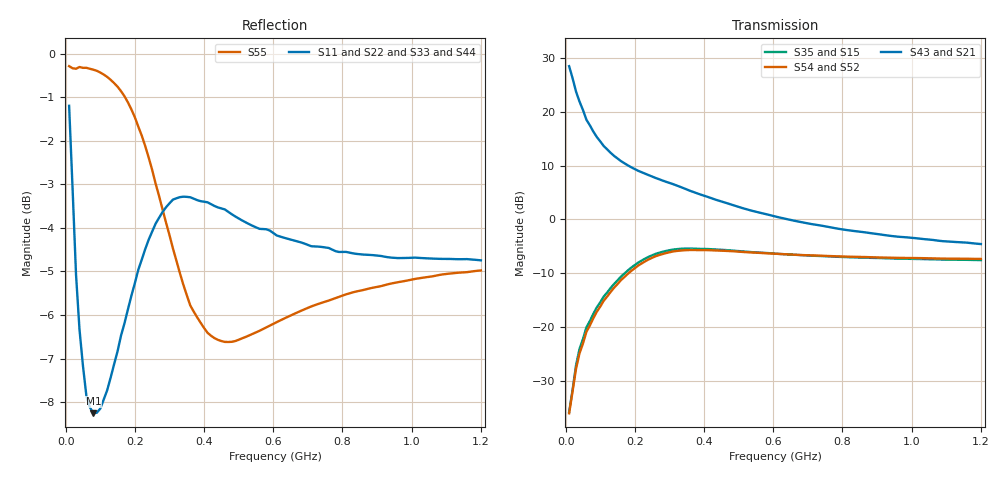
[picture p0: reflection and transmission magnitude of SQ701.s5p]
!  POLYFET RF DEVICES
!  S PARAMETERS FOR
!  SQ701 (EACH SIDE)
!  VDS=28, IDQ=200MA
! S1A1Die, Vds=28Vdc, Idq=200ma, Vgsth=2.60Vdc
! Date: Thu Jul 23 11:46:25 1998
!AWR Design Environment (2053) Wed Feb 04 15:37:27 2004
!freq-unit  param-type  data-format  keyword  impedance-ohms
# MHz  S  MA  R  50
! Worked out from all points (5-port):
!   120 points, 10 MHz to 1.2 GHz, reference 50 ohm
!   strongest paths, dB at 10 MHz, 310 MHz, 610 MHz, 910 MHz, 1.2 GHz:
!     S43: 28.5, 6.6, 0.5, -2.8, -4.6
!     S21: 28.5, 6.6, 0.5, -2.8, -4.6
!     S54: -36.0, -6.0, -6.4, -7.1, -7.4
!     S52: -36.0, -6.0, -6.4, -7.1, -7.4
!     S35: -35.8, -5.6, -6.4, -7.2, -7.6
!     S15: -35.8, -5.6, -6.4, -7.2, -7.6
!   lowest |S11| = -8.3 dB at 80 MHz (marker M1), VSWR 2.26, Z = 51.2 - j42.4 ohm
!   |S11| at or under -10 dB: nowhere
